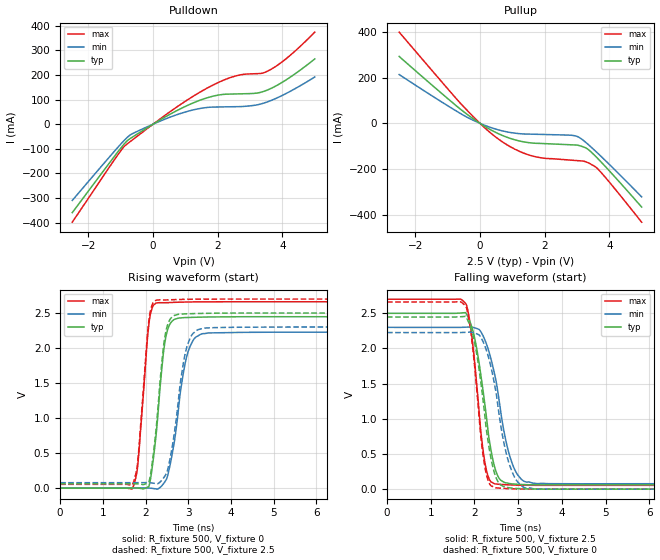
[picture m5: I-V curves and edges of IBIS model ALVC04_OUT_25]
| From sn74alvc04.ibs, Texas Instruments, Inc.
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[Model]   ALVC04_OUT_25
Model_type  Output
Vref =   0
Rref =   500
Cref =   30p
Vmeas =   1.25
| variable   typ   min   max
C_comp   6.30pF   4.36pF   8.32pF
| C_pullup   6.73pF   5.62pF   8.00pF
| C_pulldown   5.88pF   4.36pF   8.32pF
[Temperature Range]   40   100   -40
| Ambient temperature   25   85   -40
[Voltage range]   2.5   2.3   2.7
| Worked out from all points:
|   slope of the pulldown table from 0 to 0.375 V, typ, clamps not added: 12.8 ohm
|   slope of the pullup table from 0 to 0.375 V, typ, clamps not added: 11.8 ohm
|   rising waveform, R_fixture 500, V_fixture 0: 20-80 % time 228ps typ, 316ps min, 196ps max; typ from 0 V to 2.45 V
|   falling waveform, R_fixture 500, V_fixture 2.5: 20-80 % time 333ps typ, 407ps min, 250ps max; typ from 2.5 V to 0.061 V
|   rising waveform, R_fixture 500, V_fixture 2.5: 20-80 % time 224ps typ, 302ps min, 194ps max; typ from 0.061 V to 2.5 V
|   falling waveform, R_fixture 500, V_fixture 0: 20-80 % time 321ps typ, 394ps min, 248ps max; typ from 2.45 V to 0 V
[Pulldown]
| ALVC04_OUT_25
|   Voltage   I(typ)   I(min)   I(max)
-2.5V     -359.5mA   -309.9mA   -398.3mA
-1.005V   -98.29mA   -81.75mA   -109mA
-805mV    -68.14mA   -54.37mA   -80.71mA
-595mV    -48.81mA   -35.8mA    -59.5mA
815mV     60.4mA     41.95mA    77.05mA
1.84V     113.2mA    69.38mA    158mA
2.53V     122.7mA    70.94mA    195mA
3.1V      124.8mA    75.93mA    204.6mA
3.39V     131.8mA    84.2mA     207.5mA
3.675V    147mA      97.61mA    225mA
4.255V    192.1mA    134.3mA    281.3mA
5V        264.9mA    191.7mA    374.1mA
[Pullup]
| ALVC04_OUT_25
|   Voltage   I(typ)   I(min)   I(max)
-2.5V     292.7mA    213.6mA    399.4mA
-570mV    57.93mA    40.21mA    82.66mA
40mV      -3.736mA   -2.447mA   -5.503mA
440mV     -36.5mA    -23.23mA   -54.89mA
1V        -68.84mA   -41.49mA   -107.4mA
1.56V     -85.45mA   -47.34mA   -140.5mA
1.985V    -88.74mA   -48.85mA   -152.7mA
2.815V    -93.95mA   -52.11mA   -161.1mA
3.03V     -96.06mA   -58.95mA   -163.4mA
3.315V    -111.2mA   -88.55mA   -170.7mA
3.635V    -152.9mA   -129.9mA   -198.3mA
5V        -366.4mA   -321.9mA   -432.8mA
[Ramp]
| ALVC04_OUT_25
| variable   typ   min   max
dV/dt_r   1.48/2.34E-10   1.35/3.20E-10   1.61/2.03E-10
dV/dt_f   1.47/3.49E-10   1.34/4.28E-10   1.59/2.60E-10
R_load = 500
[Rising Waveform]
| ALVC04_OUT_25
R_fixture =   500
C_fixture =   0
L_fixture =   0
V_fixture =   0
V_fixture_min = 0
V_fixture_max = 0
|   Time   V(typ)   V(min)   V(max)
0s        34.14pV    4.276nV    26.61pV
1.695ns   578.5uV    309.9uV    -2.872mV
1.82ns    55.86uV    669.7uV    338.1mV
2.085ns   33.13mV    603.8uV    2.371V
2.265ns   868.4mV    -14.19mV   2.646V
2.42ns    1.931V     60.63mV    2.648V
2.56ns    2.329V     284.8mV    2.65V
2.985ns   2.437V     1.923V     2.658V
3.48ns    2.444V     2.216V     2.661V
40ns      2.447V     2.226V     2.661V
[Falling Waveform]
| ALVC04_OUT_25
R_fixture =   500
C_fixture =   0
L_fixture =   0
V_fixture =   2.5
V_fixture_min = 2.3
V_fixture_max = 2.7
|   Time   V(typ)   V(min)   V(max)
0s        2.5V       2.3V       2.7V
1.815ns   2.491V     2.303V     2.624V
2.015ns   2.115V     2.291V     1.736V
2.23ns    1.241V     2.133V     409.8mV
2.34ns    692.9mV    1.935V     138.8mV
2.48ns    274mV      1.577V     72.9mV
2.695ns   92.57mV    756.6mV    62.83mV
2.88ns    73.15mV    335.7mV    57.86mV
3.415ns   60.8mV     78.67mV    53.4mV
40ns      60.54mV    76.61mV    53.33mV
[Rising Waveform]
| ALVC04_OUT_25
R_fixture =   500
C_fixture =   0
L_fixture =   0
V_fixture =   2.5
V_fixture_min = 2.3
V_fixture_max = 2.7
|   Time   V(typ)   V(min)   V(max)
0s        60.54mV    76.61mV    53.33mV
1.695ns   60.99mV    76.84mV    50.75mV
1.82ns    60.39mV    77.11mV    393.8mV
2.085ns   95.16mV    76.77mV    2.424V
2.265ns   953.3mV    62.3mV     2.686V
2.415ns   1.989V     136.7mV    2.687V
2.535ns   2.361V     304.4mV    2.689V
2.955ns   2.49V      1.984V     2.697V
3.395ns   2.496V     2.286V     2.7V
40ns      2.5V       2.3V       2.7V
[Falling Waveform]
| ALVC04_OUT_25
R_fixture =   500
C_fixture =   0
L_fixture =   0
V_fixture =   0
V_fixture_min = 0
V_fixture_max = 0
|   Time   V(typ)   V(min)   V(max)
0s        2.447V     2.226V     2.661V
1.815ns   2.437V     2.23V      2.583V
2.015ns   2.045V     2.216V     1.672V
2.225ns   1.11V      2.054V     363mV
2.335ns   585.1mV    1.843V     87.58mV
2.48ns    185.2mV    1.419V     18.53mV
2.67ns    35.6mV     666.6mV    9.845mV
2.865ns   13.52mV    239.2mV    4.545mV
3.415ns   268.5uV    440.7uV    48.31uV
40ns      33.76pV    4.276nV    26.2pV
